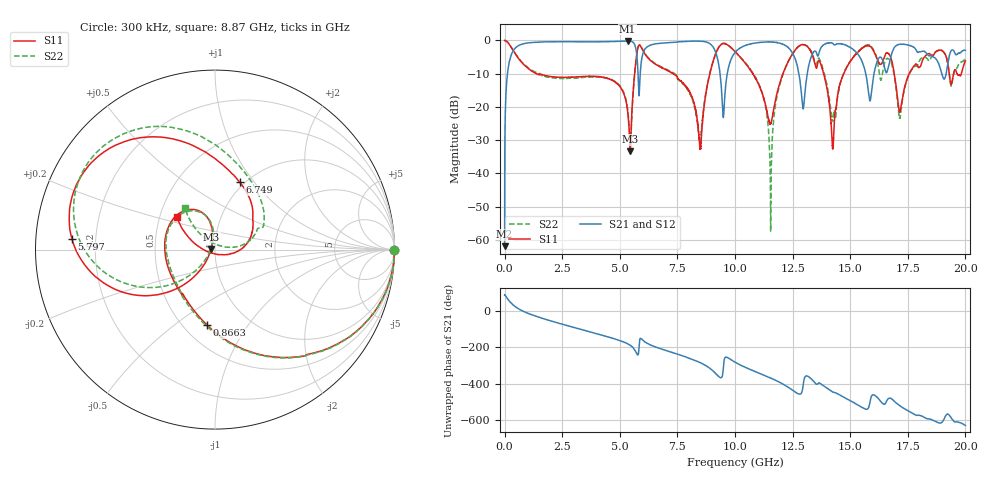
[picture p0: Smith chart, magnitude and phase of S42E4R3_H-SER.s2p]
! Created Wed Nov 25 21:45:36 2020
# khz S ma R 50
! 2 Port Network Data from SP1.SP block
! freq  magS11  angS11  magS21  angS21  magS12  angS12  magS22  angS22
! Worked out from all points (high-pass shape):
!   20001 points, 300 kHz to 20 GHz, reference 50 ohm
!   highest |S21| = -0.18 dB at 5.334 GHz (marker M1); lowest = -61.9 dB at 300 kHz (marker M2)
!   |S21| within 3 dB of the highest: 366.7 MHz to 5.716 GHz (5.349 GHz wide, 176 % of centre); 6.046 GHz to 9.141 GHz (3.095 GHz wide, 40.8 % of centre)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
!   lowest |S11| = -33.3 dB at 5.456 GHz (marker M3), VSWR 1.04, Z = 47.9 + j0.303 ohm
!   |S11| at or under -10 dB: 1.384 GHz to 5.644 GHz (4.26 GHz wide, 121 % of centre); 7.319 GHz to 8.908 GHz (1.589 GHz wide, 19.6 % of centre); 10.77 GHz to 12.08 GHz (1.311 GHz wide, 11.5 % of centre)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
!   |S22| runs from -57.4 to 0.0 dB; largest |S21 - S12| = 0.018
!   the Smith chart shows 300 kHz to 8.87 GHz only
!   S11 on the Smith chart (normalised r, x): 300 kHz: open; 866.3 MHz: 0.65, -0.66; 5.797 GHz: 0.11, +0.04; 6.749 GHz: 0.95, +0.85; 8.87 GHz: 0.62, +0.24
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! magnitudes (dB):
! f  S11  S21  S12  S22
! 300 kHz  0.0  -61.9  -61.4  0.0
! 177.3 MHz  -0.9  -7.4  -7.3  -0.9
! 866.3 MHz  -7.5  -0.9  -0.9  -7.4
! 3.334 GHz  -10.9  -0.4  -0.4  -11.1
! 5.334 GHz  -20.9  -0.2  -0.2  -20.3
! 5.456 GHz  -33.3  -0.2  -0.2  -32.5
! 5.797 GHz  -1.9  -11.0  -11.0  -1.9
! 6.667 GHz  -7.6  -0.9  -0.9  -7.4
! 6.749 GHz  -7.9  -0.9  -0.9  -7.7
! 8.48 GHz  -32.1  -0.2  -0.2  -30.8
! 8.87 GHz  -11.1  -0.8  -0.8  -10.9
! 9.496 GHz  -0.9  -23.2  -23.3  -0.9
! 10 GHz  -3.3  -3.6  -3.7  -3.3
! 11.55 GHz  -25.0  -0.5  -0.5  -51.7
! 12.18 GHz  -8.4  -1.5  -1.4  -8.5
! 12.95 GHz  -1.2  -20.5  -20.4  -1.3
! 13.33 GHz  -3.9  -4.5  -4.5  -3.7
! 14.24 GHz  -32.5  -0.9  -0.9  -24.2
! 15.06 GHz  -5.8  -2.4  -2.4  -5.6
! 16.67 GHz  -3.9  -7.7  -7.8  -5.6
! 17.16 GHz  -21.5  -1.1  -1.2  -23.3
! 20 GHz  -6.1  -3.0  -3.0  -5.6
